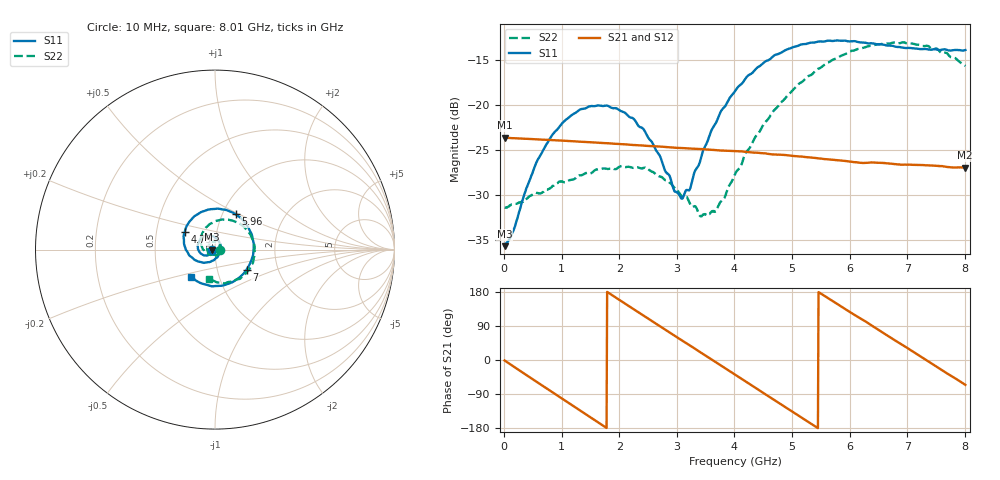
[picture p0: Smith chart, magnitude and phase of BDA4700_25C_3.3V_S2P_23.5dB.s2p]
!Agilent Technologies,E5071B,MY42404982,A.09.10
!Date: Mon Oct 20 18:12:56 2025
!Data & Calibration Information:
!Freq	S11:SOLT2(ON)	S21:SOLT2(ON)	S12:SOLT2(ON)	S22:SOLT2(ON)
# Hz S RI R 50
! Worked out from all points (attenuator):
!   801 points, 10 MHz to 8.01 GHz, reference 50 ohm
!   highest |S21| = -23.57 dB at 10 MHz (marker M1); lowest = -26.9 dB at 8 GHz (marker M2)
!   lowest |S11| = -35.6 dB at 10 MHz (marker M3), VSWR 1.03, Z = 48.4 - j0.103 ohm
!   |S11| at or under -10 dB: start of sweep to end of sweep
!   |S22| runs from -32.3 to -13.0 dB; largest |S21 - S12| = 0.00078
!   S11 on the Smith chart (normalised r, x): 10 MHz: 0.97, -0.00; 4.79 GHz: 0.70, +0.14; 5.96 GHz: 1.15, +0.48; 7 GHz: 1.38, -0.32; 8.01 GHz: 0.74, -0.24
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1e7  -0.0165 -0.00106  0.0663 -0.00141  0.0663 -0.00149  0.0271 -0.000798
1.5e8  -0.0174 -0.0093  0.0634 -0.0176  0.0633 -0.0177  0.0272 -0.00734
3.9e8  -0.0255 -0.0238  0.05 -0.042  0.05 -0.0419  0.0217 -0.0211
7e8  -0.0477 -0.033  0.0207 -0.0611  0.0207 -0.061  0.0061 -0.033
1.35e9  -0.0955 0.0048  -0.0455 -0.0433  -0.0455 -0.0433  -0.0368 -0.0181
2.08e9  -0.0526 0.0753  -0.0531 0.0295  -0.0532 0.0296  -0.0299 0.0343
2.42e9  -0.00812 0.0735  -0.0275 0.0532  -0.0274 0.0531  -0.00452 0.0446
2.68e9  0.0197 0.0502  -0.00182 0.0591  -0.00186 0.0591  0.0136 0.0381
2.96e9  0.0312 0.0117  0.0252 0.0525  0.0252 0.0524  0.0265 0.0227
3.1e9  0.029 -0.00923  0.0369 0.0447  0.0366 0.0449  0.0292 0.0111
3.23e9  0.0216 -0.0269  0.0454 0.0355  0.0455 0.0354  0.0282 0.00203
3.55e9  -0.0169 -0.0632  0.0564 0.00652  0.0565 0.00644  0.0128 -0.0209
3.7e9  -0.0432 -0.0705  0.0558 -0.00784  0.0559 -0.00805  -8.22e-05 -0.0266
4.01e9  -0.1027 -0.0619  0.0437 -0.0347  0.0437 -0.0346  -0.0318 -0.0264
4.79e9  -0.1694 0.0959  -0.0227 -0.0482  -0.0223 -0.0484  -0.0786 0.0649
5.35e9  -0.069 0.2121  -0.0505 -0.00884  -0.0504 -0.00917  -0.0158 0.148
5.96e9  0.1147 0.1963  -0.032 0.0371  -0.0322 0.0369  0.1232 0.1512
6.68e9  0.2145 -0.0101  0.0222 0.042  0.0224 0.0421  0.2205 -0.0012
7e9  0.1758 -0.1119  0.0398 0.0248  0.0399 0.0245  0.2029 -0.0868
7.49e9  0.0363 -0.2015  0.0445 -0.0125  0.0445 -0.0125  0.1028 -0.1796
8e9  -0.1287 -0.156  0.0192 -0.0408  0.0194 -0.0409  -0.0296 -0.1637
8.01e9  -0.1313 -0.1546  0.0186 -0.0412  0.0187 -0.0411  -0.0319 -0.1622
